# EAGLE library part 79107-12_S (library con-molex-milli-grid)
RECEPTACAL
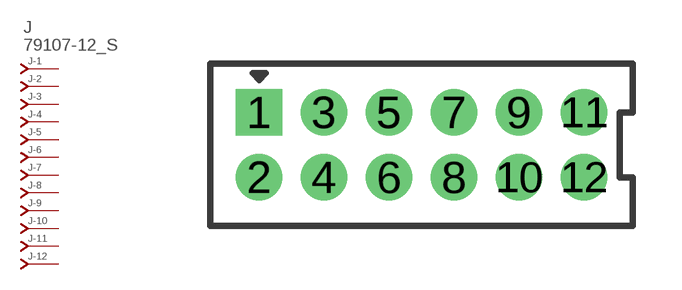
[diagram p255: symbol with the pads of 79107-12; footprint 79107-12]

Designator prefix J; gates -1=J-NV -2=J-N -3=J-N -4=J-N -5=J-N -6=J-N -7=J-N -8=J-N -9=J-N -10=J-N -11=J-N -12=J-N

## 79107-12_S  [79107-12]
1  -1:J  pas
2  -2:J  pas
3  -3:J  pas
4  -4:J  pas
5  -5:J  pas
6  -6:J  pas
7  -7:J  pas
8  -8:J  pas
9  -9:J  pas
10  -10:J  pas
11  -11:J  pas
12  -12:J  pas

## Footprint 79107-12 (pad centres in mm)
RECEPTACAL Dual Row, Vertical, Through-Hole
drill 0.914 square: 1 -5,1
drill 0.914: 2 -5,-1; 3 -3,1; 4 -3,-1; 5 -1,1; 6 -1,-1; 7 1,1; 8 1,-1; 9 3,1; 10 3,-1; 11 5,1; 12 5,-1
